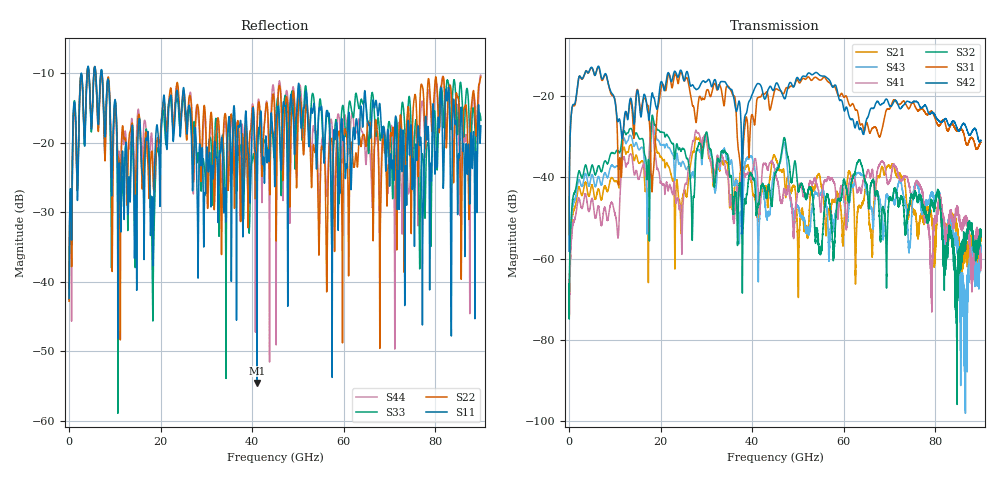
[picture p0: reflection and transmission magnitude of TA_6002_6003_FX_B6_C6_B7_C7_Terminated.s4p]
!Keysight Technologies,N5227B,US51270452,A.15.40.11
!Date: Tuesday, January 25, 2022 11:15:47
!Correction: S11(C  4-Port  )
!S12(C  4-Port  )
!S13(C  4-Port  )
!S14(C  4-Port  )
!S21(C  4-Port  )
!S22(C  4-Port  )
!S23(C  4-Port  )
!S24(C  4-Port  )
!S31(C  4-Port  )
!S32(C  4-Port  )
!S33(C  4-Port  )
!S34(C  4-Port  )
!S41(C  4-Port  )
!S42(C  4-Port  )
!S43(C  4-Port  )
!S44(C  4-Port  )
!S4P File: Measurements: <S11,S12,S13,S14>,
!<S21,S22,S23,S24>,
!<S31,S32,S33,S34>,
!<S41,S42,S43,S44>:
# Hz S  dB  R 50
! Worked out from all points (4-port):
!   9000 points, 10 MHz to 90 GHz, reference 50 ohm
!   strongest paths, dB at 10 MHz, 22.51 GHz, 45.01 GHz, 67.51 GHz, 90 GHz:
!     S42: -58.2, -16.1, -17.5, -21.3, -30.9
!     S31: -54.1, -18.0, -18.4, -29.3, -31.4
!     S32: -67.6, -31.6, -39.2, -44.5, -53.0
!     S41: -68.2, -43.7, -38.5, -37.7, -62.9
!     S43: -66.4, -34.0, -38.2, -44.0, -58.0
!     S21: -65.2, -40.4, -34.9, -39.8, -54.9
!   lowest |S11| = -54.6 dB at 41.06 GHz (marker M1), VSWR 1.00, Z = 49.9 + j0.175 ohm
!   |S11| at or under -10 dB: start of sweep to 3.967 GHz; 5.828 GHz to 6.934 GHz (1.106 GHz wide, 17.3 % of centre); 7.22 GHz to end of sweep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
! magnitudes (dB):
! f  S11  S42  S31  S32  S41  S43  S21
! 10 MHz  -42.4  -58.2  -54.1  -67.6  -68.2  -66.4  -65.2
! 4.84 GHz  -17.9  -12.9  -13.1  -37.6  -45.7  -39.9  -42.4
! 18.2 GHz  -28.1  -19.2  -42.5  -24.7  -26.8  -25.7  -26.3
! 21.79 GHz  -14.8  -14.3  -14.5  -30.1  -42.6  -32.7  -37.4
! 41.06 GHz  -54.6  -17.1  -20.8  -48.1  -38.0  -45.4  -49.6
! 46.98 GHz  -14.3  -20.5  -19.3  -30.3  -43.0  -31.5  -38.8
! 90 GHz  -17.6  -30.9  -31.4  -53.0  -62.9  -58.0  -54.9
